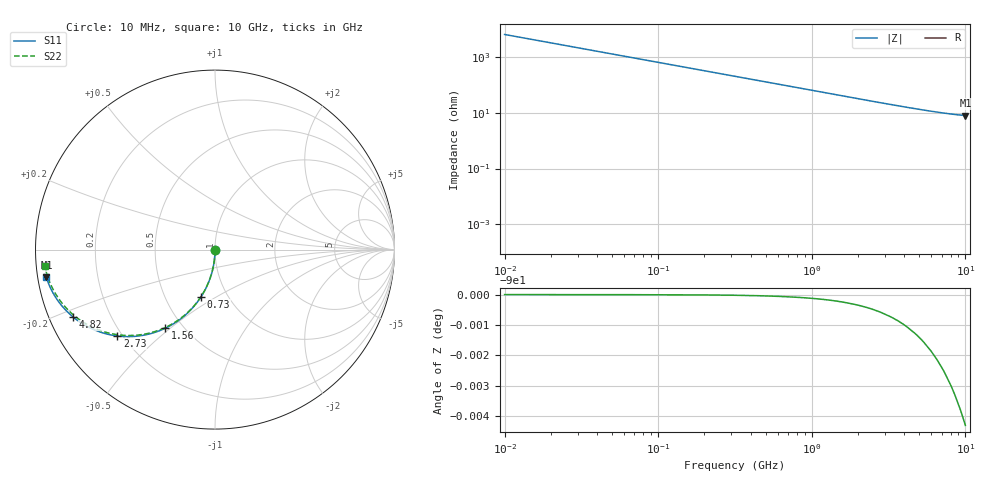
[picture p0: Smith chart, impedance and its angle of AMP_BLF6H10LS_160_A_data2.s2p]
! Created Thu Oct 06 12:07:39 2011
# ghz S ma R 50
! 2 Port Network Data from SP1.SP block
! freq  magS11  angS11  magS21  angS21  magS12  angS12  magS22  angS22
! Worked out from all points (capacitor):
!   1000 points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, 10 MHz to 10 GHz, reference 50 ohm
!   read as one part in shunt: C = 2.53 pF near 60 MHz
!   lowest |Z| = 7.87 ohm at 10 GHz (marker M1)
!   S11 on the Smith chart (normalised r, x): 10 MHz: 1.00, -0.01; 730 MHz: 0.75, -0.43; 1.56 GHz: 0.40, -0.48; 2.73 GHz: 0.18, -0.37; 4.82 GHz: 0.07, -0.22; 10 GHz: 0.02, -0.08
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0.01  0.003905 -90.2  1 -0.2  1 -0.2  0.003905 -90.2
0.04  0.01562 -90.9  0.9999 -0.9  0.9999 -0.9  0.01562 -90.9
0.07  0.02733 -91.6  0.9996 -1.6  0.9996 -1.6  0.02733 -91.6
0.09  0.03513 -92.1  0.9994 -2.1  0.9994 -2.1  0.03513 -92.1
0.11  0.04293 -92.5  0.9991 -2.6  0.9991 -2.6  0.04293 -92.6
0.14  0.0546 -93.2  0.9985 -3.2  0.9985 -3.2  0.0546 -93.3
0.2  0.07789 -94.6  0.997 -4.6  0.997 -4.6  0.07789 -94.7
0.29  0.1126 -96.7  0.9936 -6.7  0.9936 -6.7  0.1126 -96.7
0.41  0.1582 -99.4  0.9874 -9.4  0.9874 -9.4  0.1582 -99.5
0.56  0.2137 -102.7  0.9769 -12.8  0.9769 -12.8  0.2137 -102.9
0.73  0.2742 -106.4  0.9617 -16.5  0.9617 -16.5  0.2742 -106.6
1.1  0.3946 -114.0  0.9188 -24.2  0.9188 -24.2  0.3946 -114.3
1.56  0.5197 -122.4  0.8544 -32.6  0.8544 -32.6  0.5197 -122.9
1.68  0.5478 -124.4  0.8366 -34.6  0.8366 -34.6  0.5478 -124.9
2.16  0.643 -131.5  0.7659 -41.9  0.7659 -41.9  0.643 -132.2
2.73  0.7262 -138.5  0.6875 -48.9  0.6875 -48.9  0.7262 -139.3
3.34  0.7888 -144.4  0.6146 -55.0  0.6146 -55.0  0.7888 -145.5
4.82  0.875 -154.6  0.4841 -65.3  0.4841 -65.3  0.875 -156.1
5.01  0.8819 -155.5  0.4714 -66.4  0.4714 -66.4  0.8819 -157.2
6.67  0.9221 -162.3  0.3868 -73.4  0.3868 -73.4  0.9221 -164.6
8.34  0.9419 -167.1  0.3357 -78.5  0.3357 -78.5  0.9419 -170.0
10  0.952 -170.7  0.3059 -82.5  0.3059 -82.5  0.952 -174.3
